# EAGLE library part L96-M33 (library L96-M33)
Navigation BeiDou, Galileo, GLONASS, GPS, GNSS Transceiver Module 1.561GHz, 1.575GHz, 1.602GHz Integrated, Chip Surface Mount Source: Datasheet
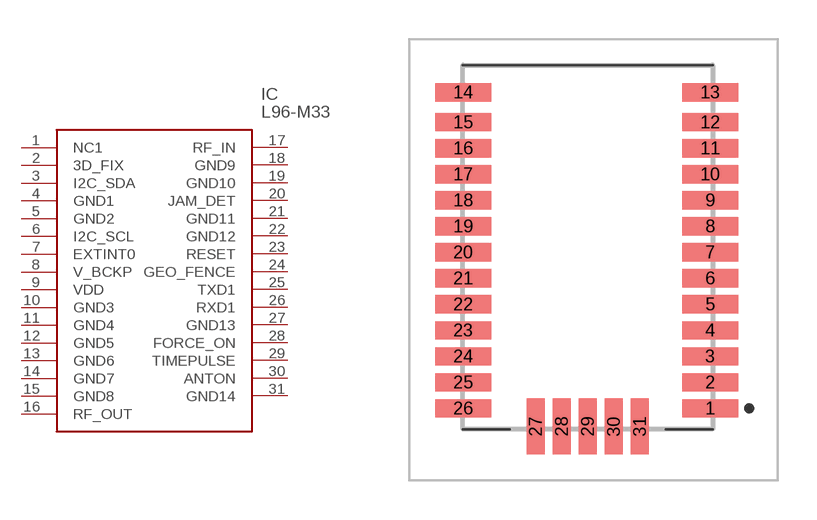
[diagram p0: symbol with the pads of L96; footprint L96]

Designator prefix IC

## L96-M33 (Arrow_Part_Number: L96-M33; Arrow_Price-Stock: https://www.arrow.com/en/products/l96-m33/quectel-wireless-solutions-co-ltd?utm_currency=USD&region=nac; Description: Navigation BeiDou, Galileo, GLONASS, GPS, GNSS Transceiver Module 1.561GHz, 1.575GHz, 1.602GHz Integrated, Chip Surface Mount; Height: mm; Manufacturer_Name: Quectel; Manufacturer_Part_Number: L96-M33; Mouser_Part_Number: 277-L96-M33; Mouser_Price-Stock: https://www.mouser.co.uk/ProductDetail/Quectel/L96-M33?qs=GedFDFLaBXHZlDfU1tecmQ%3D%3D)  [L96]
1  NC1
2  3D_FIX
3  I2C_SDA
4  GND1
5  GND2
6  I2C_SCL
7  EXTINT0
8  V_BCKP
9  VDD
10  GND3
11  GND4
12  GND5
13  GND6
14  GND7
15  GND8
16  RF_OUT
17  RF_IN
18  GND9
19  GND10
20  JAM_DET
21  GND11
22  GND12
23  RESET
24  GEO_FENCE
25  TXD1
26  RXD1
27  GND13
28  FORCE_ON
29  TIMEPULSE
30  ANTON
31  GND14

## Footprint L96 (pad centres in mm)
L96_1
smd 2.15 x 0.7: 1 4.746,-5.714; 2 4.746,-4.714; 3 4.746,-3.713; 4 4.746,-2.713; 5 4.746,-1.713; 6 4.746,-0.713; 7 4.746,0.287; 8 4.746,1.287; 9 4.746,2.287; 10 4.746,3.287; 11 4.746,4.287; 12 4.746,5.287; 13 4.746,6.438; 14 -4.744,6.438; 15 -4.744,5.287; 16 -4.744,4.287; 17 -4.744,3.287; 18 -4.744,2.287; 19 -4.744,1.287; 20 -4.744,0.287; 21 -4.744,-0.713; 22 -4.744,-1.713; 23 -4.744,-2.713; 24 -4.744,-3.713; 25 -4.744,-4.714; 26 -4.744,-5.714
smd 0.7 x 2.15: 27 -1.954,-6.412; 28 -0.954,-6.412; 29 0.046,-6.412; 30 1.046,-6.412; 31 2.046,-6.412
